(* Logix 5000 AddOnInstructionDefinition export Banner_K50_Select_Sensor_PD_v4; software revision 33.03 *)

TYPE Banner_K50Select_Coarse_Distance_v4 :
STRUCT
   PDI_Output_State : SINT;   // 0=Inactive, 1=Active. Related parameters defined in output and touch settings parameter data.
   PDI_State : SINT;   // 0=State1, 1=State2, 2=State3, 3=State4, 4=State5, 5=Out of Range. Related paraemter define din four state full logic/multicolor parameter data.
   PDI_Distance : DINT;   // Measured distance in millimeters.
END_STRUCT
END_TYPE

TYPE Banner_K50Select_Distance_4State_v4 :   // Process Data for Four State Mode.
STRUCT
   PDI_Output_State : SINT;   // 0=Inactive, 1=Active. Related parameters defined in output and touch settings parameter data.
   PDI_State : SINT;   // 0=State1, 1=State2, 2=State3, 3=State4. Related parameters defined in four state full logic/multicolor parameter data.
   PDI_Distance : DINT;   // Measured distance in millimeters.
   PDO_Job_Control : SINT;   // 0 = Off, 1 = On.
END_STRUCT
END_TYPE

TYPE Banner_K50Select_Distance_Adv_v4 :   // Advanced Process Data information.
STRUCT
   PDI_Output_Status : SINT;   // 0 = Inactive, 1 = Active. Related parameters defined in output and touch settings parameter data.
   PDI_Distance : DINT;   // Measured distance in millimeters.
   Type : SINT;   // 0 = Off, 1 = Steady, 2 = Flash, 3 = Two Color Flash, 4 = 50/50, 5 = 50/50 Rotate, 6 = Chase, 7 = Intensity Sweep, 8 = Sequence.
   Direction : SINT;   // 0 = CCW, 1 = CW.
   Pattern : SINT;   // 0 = Flash, 1 = Strobe, 2 = Three Pulse, 3 = SOS, 4 = Random.
   Speed : SINT;   // 0 = Slow, 1 = Medium, 2 = Fast, 3 = Custom.
   Static_Sequence : INT;   // 0 to 255. Value describing the LED position on the device.
   Sequence_Start_Location : SINT;   // 0 = LED 1, 1 = LED 2, 2 = LED 3, 3 = LED 4, 4 = LED 5, 5 = LED 6, 6 = LED 7, 7 = LED 8.
   Color_1 : SINT;   // 0 = Green, 1 = Red, 2 = Orange, 3 = Amber, 4 = Yellow, 5 = Lime Green, 6 = Spring Green, 7 = Cyan, 8 = Sky Blue, 9 = Blue, 10 = Violet, 11 = Magenta, 12 = Rose, 13 = White, 14 = Custom 1, 15 = Custom 2.
   Color_1_Intensity : SINT;   // 0 = High, 1 = Medium, 2 = Low, 3 = Off, 4 = Custom.
   Color_2 : SINT;   // 0 = Green, 1 = Red, 2 = Orange, 3 = Amber, 4 = Yellow, 5 = Lime Green, 6 = Spring Green, 7 = Cyan, 8 = Sky Blue, 9 = Blue, 10 = Violet, 11 = Magenta, 12 = Rose, 13 = White, 14 = Custom 1, 15 = Custom 2.
   Color_2_Intensity : SINT;   // 0 = High, 1 = Medium, 2 = Low, 3 = Off, 4 = Custom.
END_STRUCT
END_TYPE

TYPE Banner_K50Select_Distance_LED_v4 :   // LED Control Process Data.
STRUCT
   PDI_Output_State : SINT;   // 0 = Inactive, 1 = Active. Related parameters defined in output and touch settings parameter data.
   PDI_Distance : DINT;   // Measured distance in millimeters.
   LED_1_Color : SINT;   // 0 = Green, 1 = Red, 2 = Orange, 3 = Amber, 4 = Yellow, 5 = Lime Green, 6 = Spring Green, 7 = Cyan, 8 = Sky Blue, 9 = Blue, 10 = Violet, 11 = Magenta, 12 = Rose, 13 = White, 14 = Custom 1, 15 = Custom 2.
   LED_1_Intensity : SINT;   // 0 to 10 (0 to 100%).
   LED_2_Color : SINT;   // 0 = Green, 1 = Red, 2 = Orange, 3 = Amber, 4 = Yellow, 5 = Lime Green, 6 = Spring Green, 7 = Cyan, 8 = Sky Blue, 9 = Blue, 10 = Violet, 11 = Magenta, 12 = Rose, 13 = White, 14 = Custom 1, 15 = Custom 2.
   LED_2_Intensity : SINT;   // 0 to 10 (0 to 100%).
   LED_3_Color : SINT;   // 0 = Green, 1 = Red, 2 = Orange, 3 = Amber, 4 = Yellow, 5 = Lime Green, 6 = Spring Green, 7 = Cyan, 8 = Sky Blue, 9 = Blue, 10 = Violet, 11 = Magenta, 12 = Rose, 13 = White, 14 = Custom 1, 15 = Custom 2.
   LED_3_Intensity : SINT;   // 0 to 10 (0 to 100%).
   LED_4_Color : SINT;   // 0 = Green, 1 = Red, 2 = Orange, 3 = Amber, 4 = Yellow, 5 = Lime Green, 6 = Spring Green, 7 = Cyan, 8 = Sky Blue, 9 = Blue, 10 = Violet, 11 = Magenta, 12 = Rose, 13 = White, 14 = Custom 1, 15 = Custom 2.
   LED_4_Intensity : SINT;   // 0 to 10 (0 to 100%).
   LED_5_Color : SINT;   // 0 = Green, 1 = Red, 2 = Orange, 3 = Amber, 4 = Yellow, 5 = Lime Green, 6 = Spring Green, 7 = Cyan, 8 = Sky Blue, 9 = Blue, 10 = Violet, 11 = Magenta, 12 = Rose, 13 = White, 14 = Custom 1, 15 = Custom 2.
   LED_5_Intensity : SINT;   // 0 to 10 (0 to 100%).
   LED_6_Color : SINT;   // 0 = Green, 1 = Red, 2 = Orange, 3 = Amber, 4 = Yellow, 5 = Lime Green, 6 = Spring Green, 7 = Cyan, 8 = Sky Blue, 9 = Blue, 10 = Violet, 11 = Magenta, 12 = Rose, 13 = White, 14 = Custom 1, 15 = Custom 2.
   LED_6_Intensity : SINT;   // 0 to 10 (0 to 100%).
   LED_7_Color : SINT;   // 0 = Green, 1 = Red, 2 = Orange, 3 = Amber, 4 = Yellow, 5 = Lime Green, 6 = Spring Green, 7 = Cyan, 8 = Sky Blue, 9 = Blue, 10 = Violet, 11 = Magenta, 12 = Rose, 13 = White, 14 = Custom 1, 15 = Custom 2.
   LED_7_Intensity : SINT;   // 0 to 10 (0 to 100%).
   LED_8_Color : SINT;   // 0 = Green, 1 = Red, 2 = Orange, 3 = Amber, 4 = Yellow, 5 = Lime Green, 6 = Spring Green, 7 = Cyan, 8 = Sky Blue, 9 = Blue, 10 = Violet, 11 = Magenta, 12 = Rose, 13 = White, 14 = Custom 1, 15 = Custom 2.
   LED_8_Intensity : SINT;   // 0 to 10 (0 to 100%).
   Vibration_Feedback : SINT;   // 0 = Off, 1 = On, 2 = Pattern.
   Vibration_Pattern : SINT;   // 0 = Off, 1 = On, 2 = 3 Pulses, 3 = SOS, 4 = Random.
   Vibration_Speed : SINT;   // 0 = Slow, 1 = Medium, 2 = Fast, 3 = Custom.
END_STRUCT
END_TYPE

TYPE Banner_K50Select_Distance_MC_v4 :   // Process Data for Multicolor
STRUCT
   PDI_Out_State : SINT;   // 0=Inactive, 1=Active. Related parameters defined in output and touch settings parameter data.
   PDI_State : SINT;   // 0=State1, 1=State2, 2=State3, 3=State4, 4=State5. Related parameters defined in four state full logic/multicolor parameter data.
   PDI_Distance : DINT;   // Measured distance in millimeters.
   PDO_State : SINT;   // 0=State1, 1=State2, 2=State3, 3=State4, 4=State5. Related parameters defined in four state full logic/multicolor parameter data.
END_STRUCT
END_TYPE

TYPE Banner_K50Select_Distance_PDIO_v4 :   // UDT that records the converted prcoess data.
STRUCT
   PD_MultiColor_State : Banner_K50Select_Distance_MC_v4;   // Only active when Operation Mode set to 0. State tells the light which of the four states it should be in. 0 = State 1, 1 = State 2, 2 = State 3, 3 = State 4.
   PD_FourState_Job_Input : Banner_K50Select_Distance_4State_v4;   // Only active when Operation Mode set to 1. Job Input tells the light how it should behave. 0 - Off, 1 = ON
   PD_Advanced : Banner_K50Select_Distance_Adv_v4;   // Only active when Operation Mode set to 2.
   PD_LED : Banner_K50Select_Distance_LED_v4;   // Only active when Operation Mode set to 3.
   PD_Distance : Banner_K50Select_Distance_v4;   // Only active when Operation Mode set to 5.
   PD_Coarse_Distance : Banner_K50Select_Coarse_Distance_v4;   // Only active when Operation Mode set to 6.
   PDO_DT : SINT[8];
   PDI_DT : SINT[4];
END_STRUCT
END_TYPE

TYPE Banner_K50Select_Distance_v4 :
STRUCT
   PDI_Output_State : SINT;   // 0=Inactive, 1=Active. Related parameters defined in output and touch settings parametere data.
   PDI_Distance : DINT;   // Measured distance in millimeters.
END_STRUCT
END_TYPE

ADD_ON_INSTRUCTION Banner_K50_Select_Sensor_PD_v4   (* revision 4.0, vendor Banner Engineering *)
// Takes the raw SINT information and converts that data into actual information.
VAR_IN_OUT
   PD : Banner_K50Select_Distance_PDIO_v4; {required}
END_VAR
VAR_INPUT
   Operation_Mode : SINT; {required}   // Linked from Parameters AOI or entered manually.
   Byte_Swap : BOOL; {required}
END_VAR
VAR
   PDO_Temp : SINT[8]; {access None}
   PDI_Temp : SINT[4]; {access None}
END_VAR

ROUTINE Logic   (* ladder *)
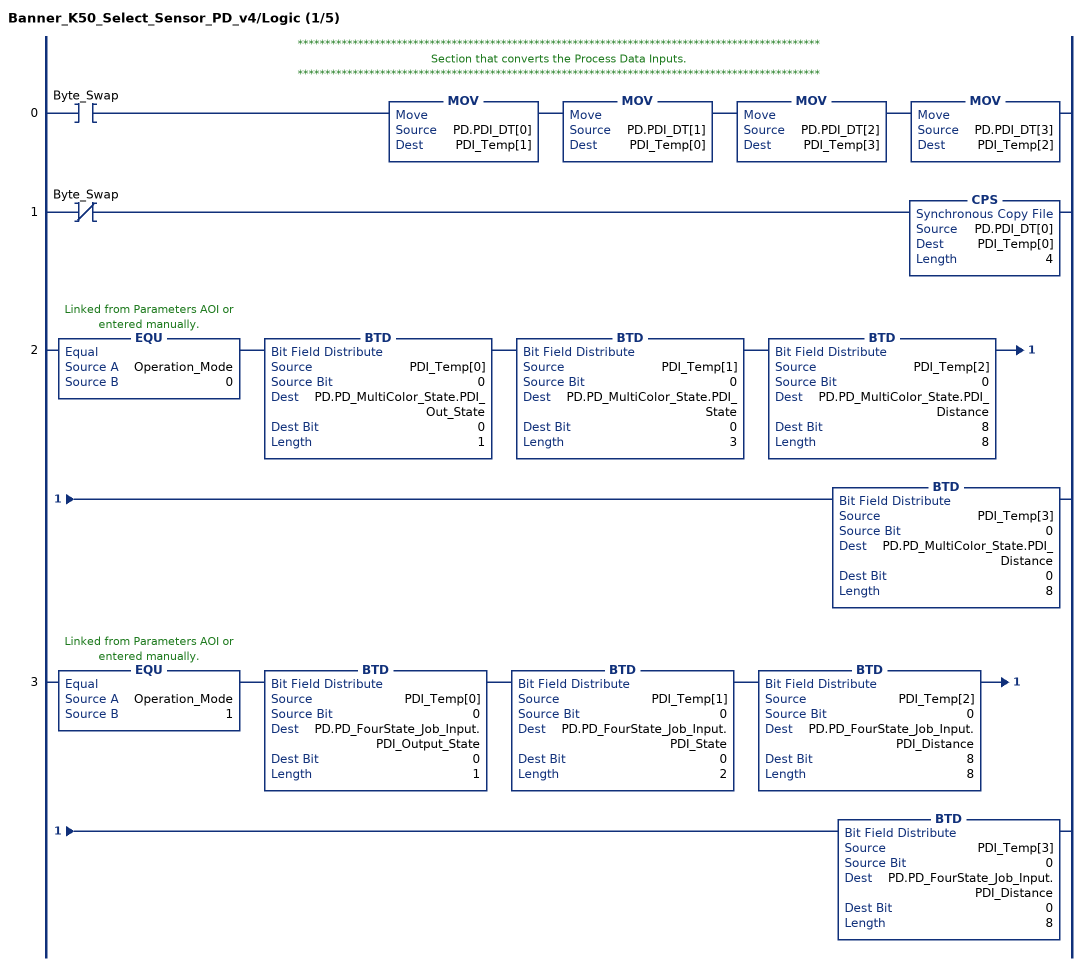
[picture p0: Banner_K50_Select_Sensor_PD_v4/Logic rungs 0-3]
   // ***********************************************************************************************
   // Section that converts the Process Data Inputs.
   // ***********************************************************************************************
   0: XIC(Byte_Swap)MOV(PD.PDI_DT[0],PDI_Temp[1])MOV(PD.PDI_DT[1],PDI_Temp[0])MOV(PD.PDI_DT[2],PDI_Temp[3])MOV(PD.PDI_DT[3],PDI_Temp[2]);
   1: XIO(Byte_Swap)CPS(PD.PDI_DT[0],PDI_Temp[0],4);
   2: EQU(Operation_Mode,0)BTD(PDI_Temp[0],0,PD.PD_MultiColor_State.PDI_Out_State,0,1)BTD(PDI_Temp[1],0,PD.PD_MultiColor_State.PDI_State,0,3)BTD(PDI_Temp[2],0,PD.PD_MultiColor_State.PDI_Distance,8,8)BTD(PDI_Temp[3],0,PD.PD_MultiColor_State.PDI_Distance,0,8);
   3: EQU(Operation_Mode,1)BTD(PDI_Temp[0],0,PD.PD_FourState_Job_Input.PDI_Output_State,0,1)BTD(PDI_Temp[1],0,PD.PD_FourState_Job_Input.PDI_State,0,2)BTD(PDI_Temp[2],0,PD.PD_FourState_Job_Input.PDI_Distance,8,8)BTD(PDI_Temp[3],0,PD.PD_FourState_Job_Input.PDI_Distance,0,8);
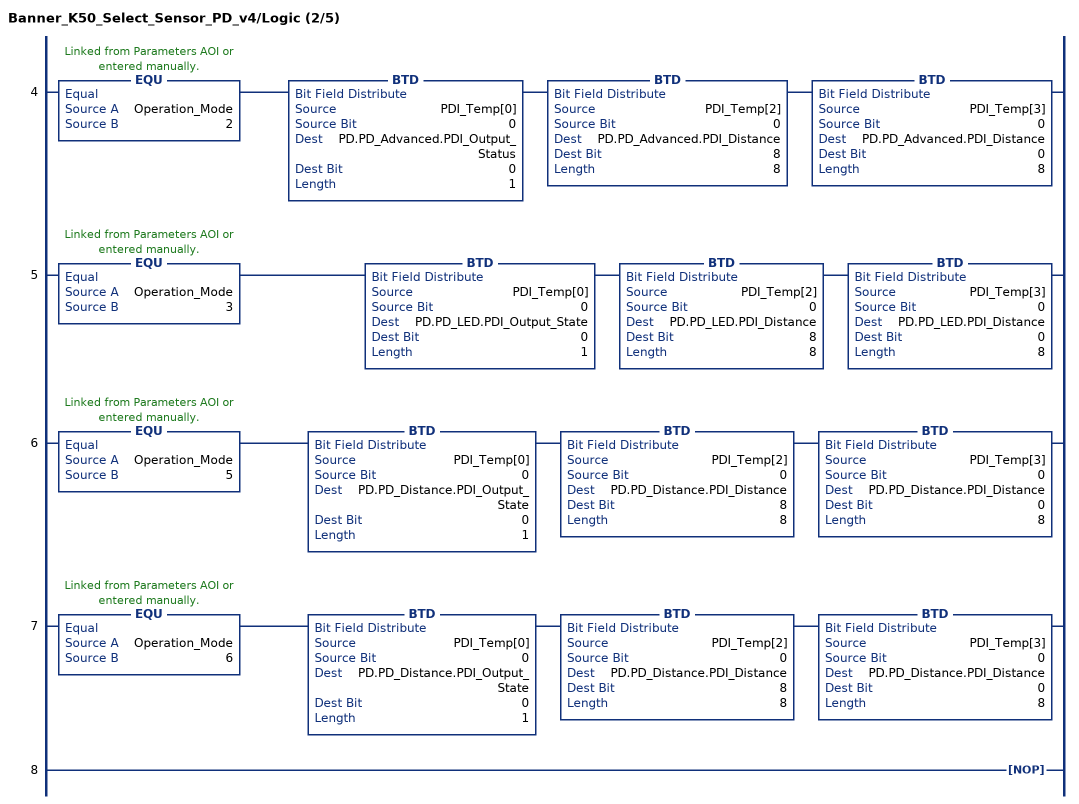
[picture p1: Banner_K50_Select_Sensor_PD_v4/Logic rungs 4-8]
   4: EQU(Operation_Mode,2)BTD(PDI_Temp[0],0,PD.PD_Advanced.PDI_Output_Status,0,1)BTD(PDI_Temp[2],0,PD.PD_Advanced.PDI_Distance,8,8)BTD(PDI_Temp[3],0,PD.PD_Advanced.PDI_Distance,0,8);
   5: EQU(Operation_Mode,3)BTD(PDI_Temp[0],0,PD.PD_LED.PDI_Output_State,0,1)BTD(PDI_Temp[2],0,PD.PD_LED.PDI_Distance,8,8)BTD(PDI_Temp[3],0,PD.PD_LED.PDI_Distance,0,8);
   6: EQU(Operation_Mode,5)BTD(PDI_Temp[0],0,PD.PD_Distance.PDI_Output_State,0,1)BTD(PDI_Temp[2],0,PD.PD_Distance.PDI_Distance,8,8)BTD(PDI_Temp[3],0,PD.PD_Distance.PDI_Distance,0,8);
   7: EQU(Operation_Mode,6)BTD(PDI_Temp[0],0,PD.PD_Distance.PDI_Output_State,0,1)BTD(PDI_Temp[2],0,PD.PD_Distance.PDI_Distance,8,8)BTD(PDI_Temp[3],0,PD.PD_Distance.PDI_Distance,0,8);
   8: NOP();
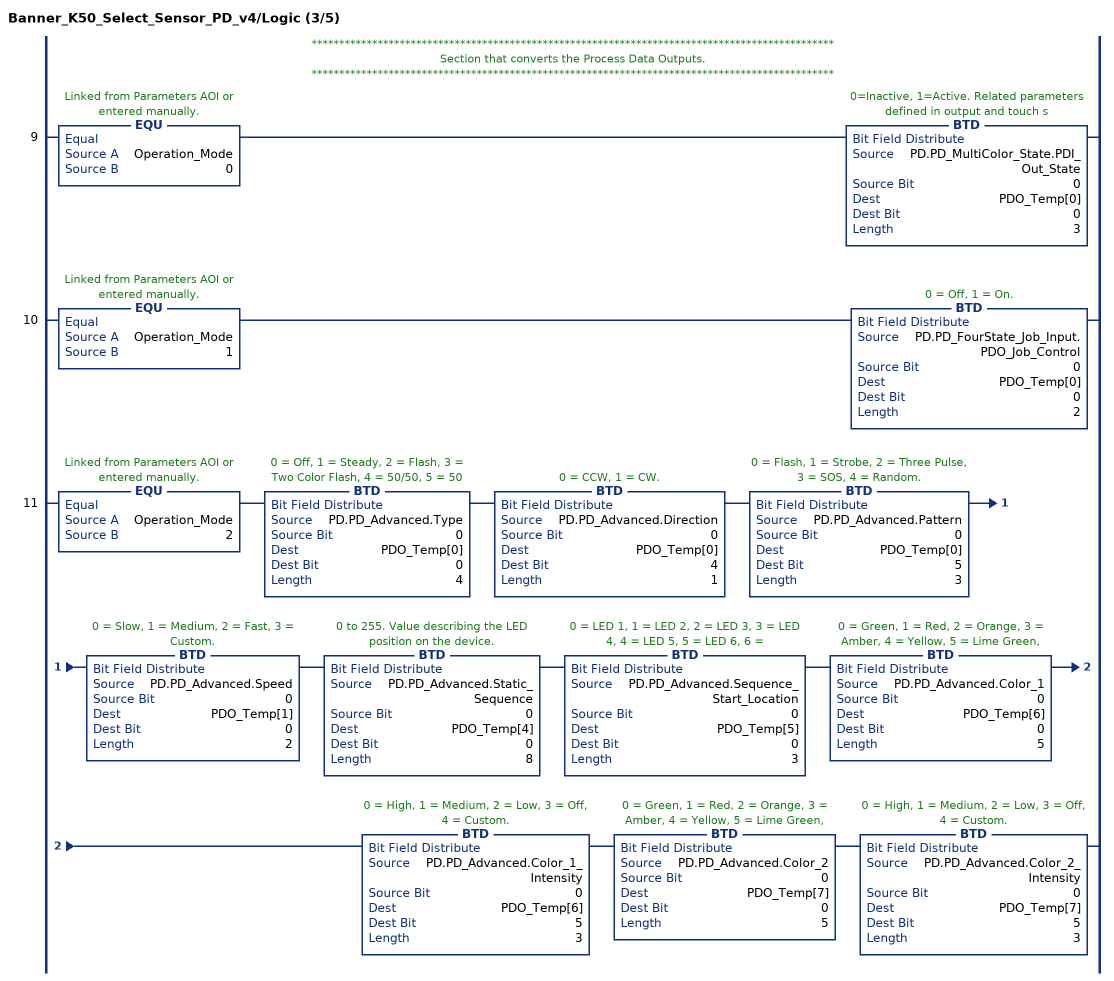
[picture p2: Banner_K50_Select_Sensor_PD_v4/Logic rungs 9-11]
   // ***********************************************************************************************
   // Section that converts the Process Data Outputs.
   // ***********************************************************************************************
   9: EQU(Operation_Mode,0)BTD(PD.PD_MultiColor_State.PDI_Out_State,0,PDO_Temp[0],0,3);
   10: EQU(Operation_Mode,1)BTD(PD.PD_FourState_Job_Input.PDO_Job_Control,0,PDO_Temp[0],0,2);
   11: EQU(Operation_Mode,2)BTD(PD.PD_Advanced.Type,0,PDO_Temp[0],0,4)BTD(PD.PD_Advanced.Direction,0,PDO_Temp[0],4,1)BTD(PD.PD_Advanced.Pattern,0,PDO_Temp[0],5,3)BTD(PD.PD_Advanced.Speed,0,PDO_Temp[1],0,2)BTD(PD.PD_Advanced.Static_Sequence,0,PDO_Temp[4],0,8)BTD(PD.PD_Advanced.Sequence_Start_Location,0,PDO_Temp[5],0,3)BTD(PD.PD_Advanced.Color_1,0,PDO_Temp[6],0,5)BTD(PD.PD_Advanced.Color_1_Intensity,0,PDO_Temp[6],5,3)BTD(PD.PD_Advanced.Color_2,0,PDO_Temp[7],0,5)BTD(PD.PD_Advanced.Color_2_Intensity,0,PDO_Temp[7],5,3);
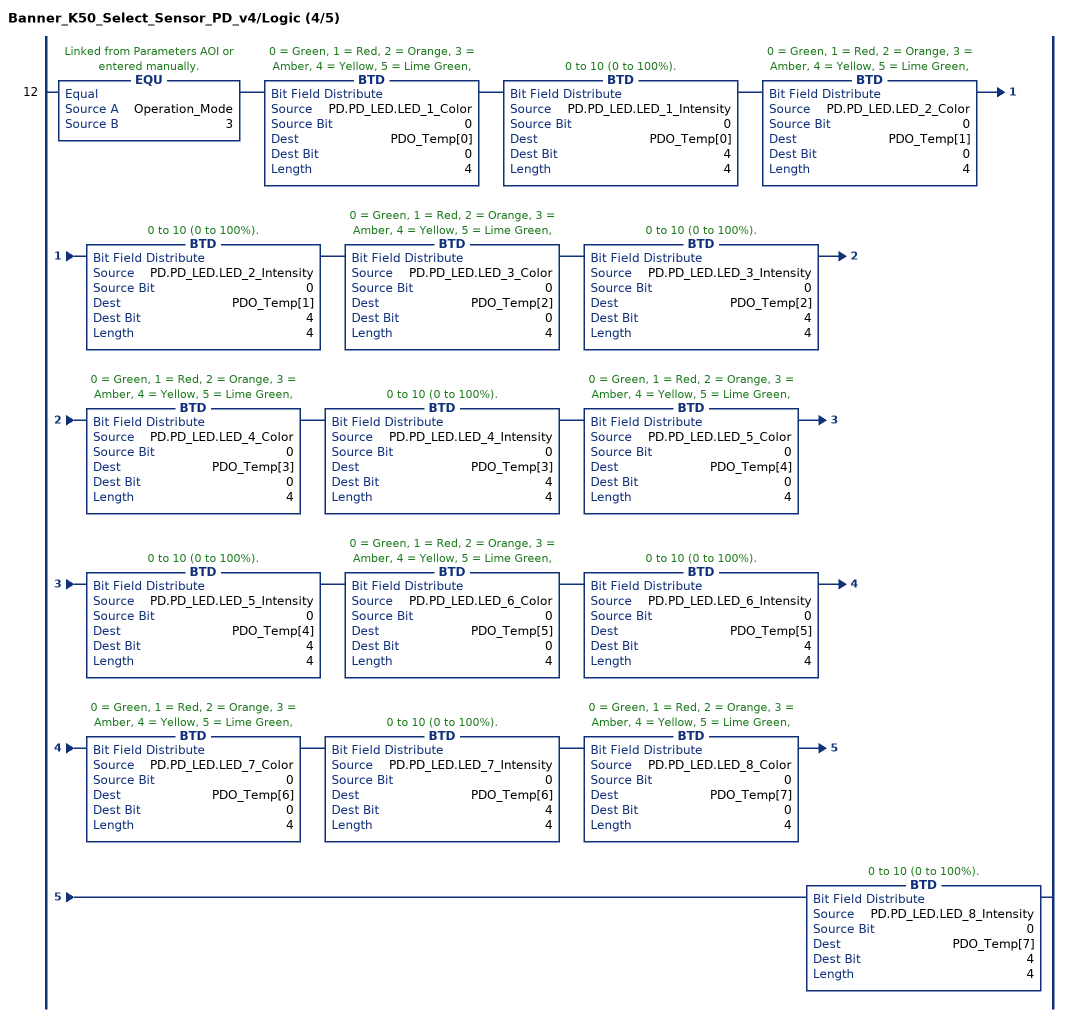
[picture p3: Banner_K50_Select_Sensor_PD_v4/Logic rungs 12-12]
   12: EQU(Operation_Mode,3)BTD(PD.PD_LED.LED_1_Color,0,PDO_Temp[0],0,4)BTD(PD.PD_LED.LED_1_Intensity,0,PDO_Temp[0],4,4)BTD(PD.PD_LED.LED_2_Color,0,PDO_Temp[1],0,4)BTD(PD.PD_LED.LED_2_Intensity,0,PDO_Temp[1],4,4)BTD(PD.PD_LED.LED_3_Color,0,PDO_Temp[2],0,4)BTD(PD.PD_LED.LED_3_Intensity,0,PDO_Temp[2],4,4)BTD(PD.PD_LED.LED_4_Color,0,PDO_Temp[3],0,4)BTD(PD.PD_LED.LED_4_Intensity,0,PDO_Temp[3],4,4)BTD(PD.PD_LED.LED_5_Color,0,PDO_Temp[4],0,4)BTD(PD.PD_LED.LED_5_Intensity,0,PDO_Temp[4],4,4)BTD(PD.PD_LED.LED_6_Color,0,PDO_Temp[5],0,4)BTD(PD.PD_LED.LED_6_Intensity,0,PDO_Temp[5],4,4)BTD(PD.PD_LED.LED_7_Color,0,PDO_Temp[6],0,4)BTD(PD.PD_LED.LED_7_Intensity,0,PDO_Temp[6],4,4)BTD(PD.PD_LED.LED_8_Color,0,PDO_Temp[7],0,4)BTD(PD.PD_LED.LED_8_Intensity,0,PDO_Temp[7],4,4);
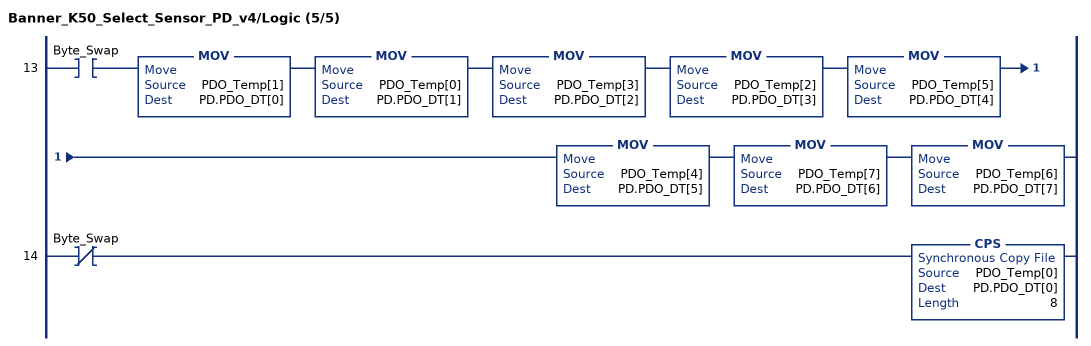
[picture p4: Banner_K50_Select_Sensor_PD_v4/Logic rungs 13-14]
   13: XIC(Byte_Swap)MOV(PDO_Temp[1],PD.PDO_DT[0])MOV(PDO_Temp[0],PD.PDO_DT[1])MOV(PDO_Temp[3],PD.PDO_DT[2])MOV(PDO_Temp[2],PD.PDO_DT[3])MOV(PDO_Temp[5],PD.PDO_DT[4])MOV(PDO_Temp[4],PD.PDO_DT[5])MOV(PDO_Temp[7],PD.PDO_DT[6])MOV(PDO_Temp[6],PD.PDO_DT[7]);
   14: XIO(Byte_Swap)CPS(PDO_Temp[0],PD.PDO_DT[0],8);
END_ROUTINE
END_ADD_ON_INSTRUCTION
